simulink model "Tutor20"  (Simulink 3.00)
settings: Solver=ode45  SolverMode=SingleTasking  StartTime=0.0  StopTime=10  RelTol=1e-3  AbsTol=1e-3
libraries: simulink3 x1

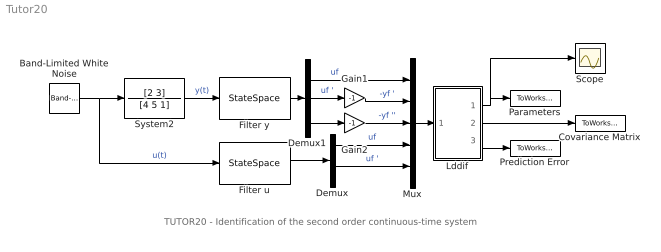
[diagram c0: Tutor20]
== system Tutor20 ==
  note: TUTOR20 - Identification of the second order continuous-time system
  Band-Limited White Noise : simulink3/Sources/Band-Limited White Noise  Cov=[0.1]  Ts=0.1  seed=[23341]
  Covariance Matrix : ToWorkspace  VariableName=CovMatrix  SampleTime=0  SaveFormat=Matrix
  Demux : Demux  Outputs=2
  Demux1 : Demux  Outputs=3
  Filter u : StateSpace  A=[0 1 0;0 0 1;-1 -3 -3]  B=[0;0;1]  C=[1 0 0;0 1 0]  D=[0;0]  X0=[0 0 0]
  Filter y : StateSpace  A=[0 1 0;0 0 1;-1 -3 -3]  B=[0;0;1]  C=eye(3)  D=[0;0;0]  X0=[0 0 0]
  Gain1 : Gain  Gain=-1  SaturateOnIntegerOverflow=on
  Gain2 : Gain  Gain=-1  SaturateOnIntegerOverflow=on
  Lddif : Subsystem  mask(LDDIF){par=[4,1], L=[0.985], d=[0.01], poc=[0 0 0 0], kov=[10e6], ts=[1]}
      mask prompts: par "No. of estimated parameters and outputs - [n,m]:"; L "Exponential forgetting - [L]:"; d "Bittanti's correction - [d]:"; poc "Initial parameter estimates - [theta(1) ... theta(n)]:"; kov "Covariance matrix (see help, standard - [10e6]):"; ts "Sampling period - [ts]:"
      mask help: LDDIF: + Bittanti's corrections Authors: Lubos Cirka and Miroslav Fikar 1998 - 2004
      mask init:
      | n=par(1); m=par(2);
  Mux : Mux  Inputs=5
  Parameters : ToWorkspace  VariableName=BA  SampleTime=0  SaveFormat=Matrix
  Prediction Error : ToWorkspace  VariableName=PredError  SampleTime=0  SaveFormat=Matrix
  Scope : Scope
  System2 : TransferFcn  Numerator=[2 3]  Denominator=[4 5 1]
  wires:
  Band-Limited White Noise/1 -> Filter u/1, System2/1  "u(t)"
  System2/1 -> Filter y/1  "y(t)"
  Demux1/2 -> Gain1/1  "uf '"
  Filter u/1 -> Demux/1
  Demux1/3 -> Gain2/1
  Filter y/1 -> Demux1/1
  Mux/1 -> Lddif/1("y, z")
  Demux/2 -> Mux/5  "uf '"
  Gain2/1 -> Mux/3  "-yf ''"
  Gain1/1 -> Mux/2  "-yf '"
  Demux1/1 -> Mux/1  "uf"
  Demux/1 -> Mux/4  "uf"
  Lddif/2(covariance matrix) -> Covariance Matrix/1
  Lddif/3(prediction error) -> Prediction Error/1
  Lddif/1(theta) -> Parameters/1, Scope/1

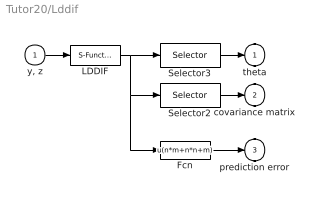
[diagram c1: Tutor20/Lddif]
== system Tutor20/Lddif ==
  "y, z" : Inport  Port=1  PortWidth=-1  SampleTime=-1  DataType=auto
  Fcn : Fcn  Expr=u(n*m+n*n+m)
  LDDIF : S-Function  FunctionName=lddif_s  Parameters=m, n, L, d, poc, kov, ts  PortCounts=[]  SFunctionModules=''
  Selector2 : Selector  Elements=[n*m:1:n*m+n*n]  InputPortWidth=n*m+n*n+m
  Selector3 : Selector  Elements=[1:1:n*m]  InputPortWidth=n*m+n*n+m
  theta : Outport  Port=1  InitialOutput=0
  covariance matrix : Outport  Port=2  InitialOutput=0
  prediction error : Outport  Port=3  InitialOutput=0
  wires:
  "y, z"/1 -> LDDIF/1
  LDDIF/1 -> Selector3/1, Selector2/1, Fcn/1
  Selector2/1 -> covariance matrix/1
  Selector3/1 -> theta/1
  Fcn/1 -> prediction error/1
